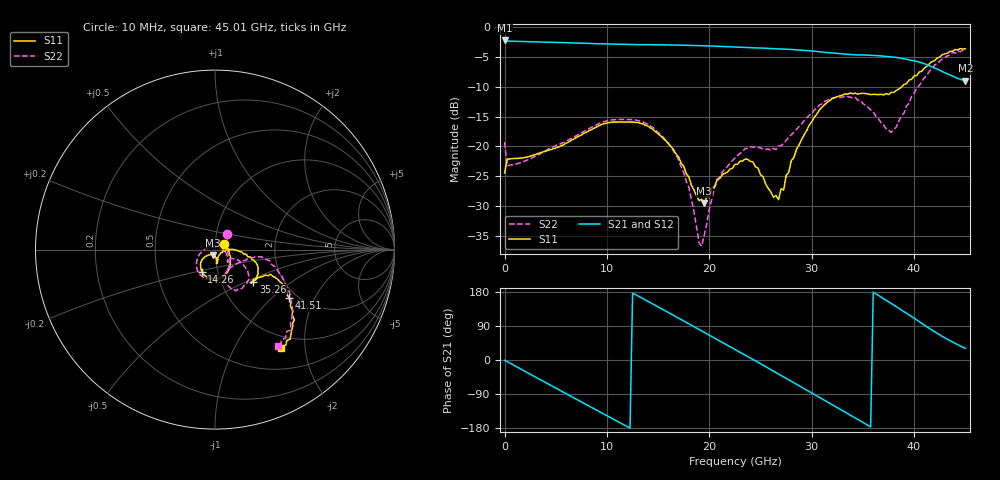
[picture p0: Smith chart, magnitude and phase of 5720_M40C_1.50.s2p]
! Device:  ADRF5720
! Description: 0.5dB LSB GaAs MMIC 6-bit Digital Attenuator
! Frequency:  0.000009 -  40 GHz
! Ports:
!	RF1	= Port 1
!	RF2	= Port 2
! Vdd:  3.3 Volt
! Vss:  -3.3 Volt
! Control:  0/3.3 Volt
! State:  1.50 dB attenuation
! Data:  The device was measured using G-S-G Probes on a matrix board.
!  Data was collected using an calibrated 4 port network analyzer.
!  The reference plane for this measurement is at the launchers.
! Note:  Analog Devices supplies this data as a sample of measured data
!  for this product.  Your particular data for this product may vary.
!  Data was taken at -40 degrees C.
!  Analog Devices reserves the right to change this data at anytime.
# GHZ S DB R 45.0
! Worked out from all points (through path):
!   181 points, 10 MHz to 45.01 GHz, reference 45 ohm
!   highest |S21| = -2.21 dB at 10 MHz (marker M1); lowest = -8.9 dB at 45.01 GHz (marker M2)
!   group delay of S21, straight-line fit = 42.4 ps
!   lowest |S11| = -29.6 dB at 19.51 GHz (marker M3), VSWR 1.07, Z = 44.1 - j2.81 ohm
!   |S11| at or under -10 dB: start of sweep to 38.78 GHz
!   |S22| runs from -36.8 to -3.9 dB; largest |S21 - S12| = 0.0029
!   S11 on the Smith chart (normalised r, x): 10 MHz: 1.11, +0.07; 14.26 GHz: 0.84, -0.21; 35.26 GHz: 1.42, -0.55; 41.51 GHz: 1.81, -1.31; 45.01 GHz: 0.81, -1.57
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0.01  -24.47 30.1  -2.21 -1.0  -2.23 -1.0  -19.27 52.8
0.26  -22.17 0.1  -2.31 -4.1  -2.33 -4.1  -23.27 0.1
4.26  -20.64 -22.9  -2.50 -63.2  -2.52 -63.2  -20.47 -28.3
7.76  -17.80 -50.8  -2.68 -114.4  -2.70 -114.4  -17.46 -58.9
11.26  -15.90 -86.6  -2.85 -165.2  -2.87 -165.2  -15.48 -96.3
14.26  -16.91 -120.8  -2.93 151.2  -2.94 151.1  -16.62 -132.3
15.26  -18.24 -131.0  -2.94 136.4  -2.96 136.3  -18.03 -145.2
17.51  -23.35 -143.5  -3.01 102.9  -3.03 102.8  -24.41 -178.9
19.01  -29.11 -124.9  -3.07 80.4  -3.09 80.3  -36.22 115.1
19.51  -29.56 -106.6  -3.11 72.9  -3.12 72.8  -34.87 47.4
20.51  -26.80 -82.0  -3.17 57.9  -3.19 57.8  -26.85 3.6
22.76  -23.00 -81.0  -3.33 24.0  -3.35 23.9  -21.52 -32.9
24.26  -22.61 -82.8  -3.44 1.5  -3.45 1.4  -20.14 -44.5
26.76  -28.95 -29.9  -3.62 -36.8  -3.64 -36.9  -19.92 -31.4
28.01  -22.42 -1.4  -3.73 -56.1  -3.75 -56.2  -18.05 -25.8
30.26  -15.09 -8.5  -4.02 -91.3  -4.05 -91.5  -13.88 -31.2
33.01  -11.39 -27.6  -4.46 -133.7  -4.49 -133.8  -11.71 -52.2
35.26  -11.12 -40.0  -4.65 -168.6  -4.68 -168.8  -13.09 -69.1
37.76  -10.93 -36.7  -4.97 149.4  -4.99 149.2  -17.65 -49.7
39.76  -8.75 -24.6  -5.53 114.7  -5.56 114.5  -11.59 -8.8
41.51  -6.09 -33.2  -6.47 83.0  -6.49 82.9  -7.36 -24.9
45.01  -3.61 -56.1  -8.95 30.6  -8.98 30.5  -3.87 -56.6
